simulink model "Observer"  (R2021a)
settings: Solver=VariableStepAuto  StartTime=0.0  StopTime=10  RelTol=1e-3
InitFcn:
  | initParams
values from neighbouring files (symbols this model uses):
  A = [-2 -2 1;0 -2 -1;0 0 -2]    [initParams.m]
  B = [0 1 1;0 0 2;1 0 0]    [initParams.m]
  C = [1 0]    [initParams.m]
  L = place(A',C',ev).'    [initParams.m]
  x0 = [0.2;0.1]    [initParams.m]
  x0s = [0;0]    [initParams.m]

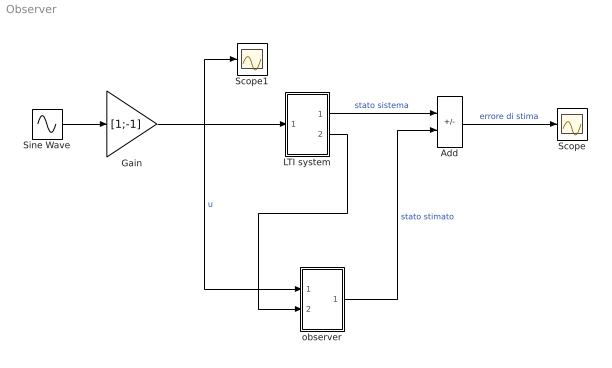
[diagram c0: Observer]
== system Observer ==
  Add : Sum  Inputs=+-
  Gain : Gain  Gain=[1;-1]
  LTI system : Subsystem
  Scope : Scope
  Scope1 : Scope
  Sine Wave : Sin  Phase=pi/2  SampleTime=0
  observer : Subsystem
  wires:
  Sine Wave/1 -> Gain/1
  LTI system/2(y) -> observer/2(y)
  LTI system/1(x) -> Add/1  "stato sistema"
  observer/1(xHat) -> Add/2  "stato stimato"
  Add/1 -> Scope/1  "errore di stima"
  Gain/1 -> Scope1/1, observer/1(u), LTI system/1(u)  "u"

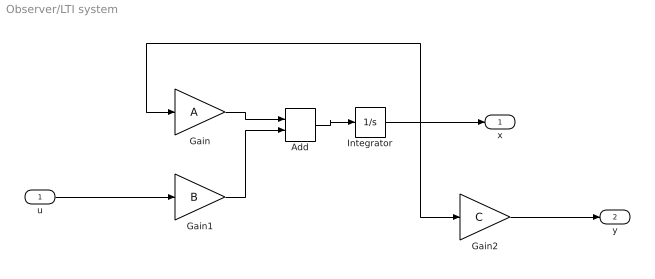
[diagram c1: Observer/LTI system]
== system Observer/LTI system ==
  u : Inport
  Add : Sum
  Gain : Gain  Gain=A  Multiplication=Matrix(K*u) (u vector)
  Gain1 : Gain  Gain=B  Multiplication=Matrix(K*u) (u vector)
  Gain2 : Gain  Gain=C  Multiplication=Matrix(K*u) (u vector)
  Integrator : Integrator  InitialCondition=x0
  x : Outport
  y : Outport  Port=2
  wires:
  Gain1/1 -> Add/2
  Integrator/1 -> x/1, Gain2/1, Gain/1
  Gain/1 -> Add/1
  Add/1 -> Integrator/1
  u/1 -> Gain1/1
  Gain2/1 -> y/1

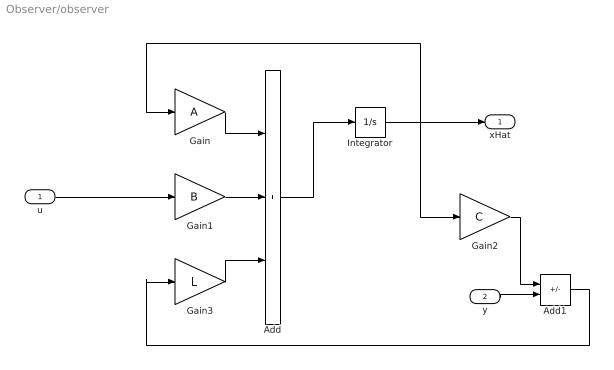
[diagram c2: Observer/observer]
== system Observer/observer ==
  u : Inport
  y : Inport  Port=2
  Add : Sum  Inputs=+++
  Add1 : Sum  Inputs=-+
  Gain : Gain  Gain=A  Multiplication=Matrix(K*u) (u vector)
  Gain1 : Gain  Gain=B  Multiplication=Matrix(K*u) (u vector)
  Gain2 : Gain  Gain=C  Multiplication=Matrix(K*u) (u vector)
  Gain3 : Gain  Gain=L  Multiplication=Matrix(K*u) (u vector)
  Integrator : Integrator  InitialCondition=x0s
  xHat : Outport
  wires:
  Gain1/1 -> Add/2
  Integrator/1 -> xHat/1, Gain2/1, Gain/1
  Gain/1 -> Add/1
  Add/1 -> Integrator/1
  u/1 -> Gain1/1
  Gain2/1 -> Add1/1
  y/1 -> Add1/2
  Gain3/1 -> Add/3
  Add1/1 -> Gain3/1
